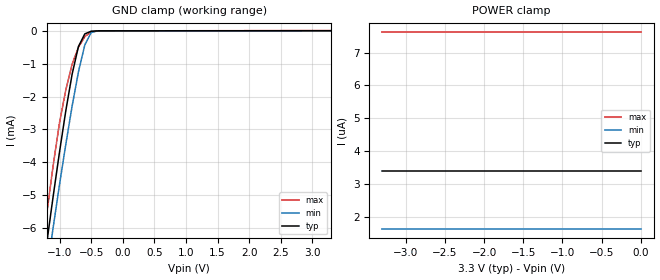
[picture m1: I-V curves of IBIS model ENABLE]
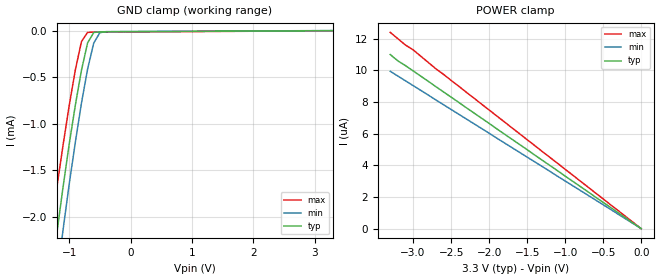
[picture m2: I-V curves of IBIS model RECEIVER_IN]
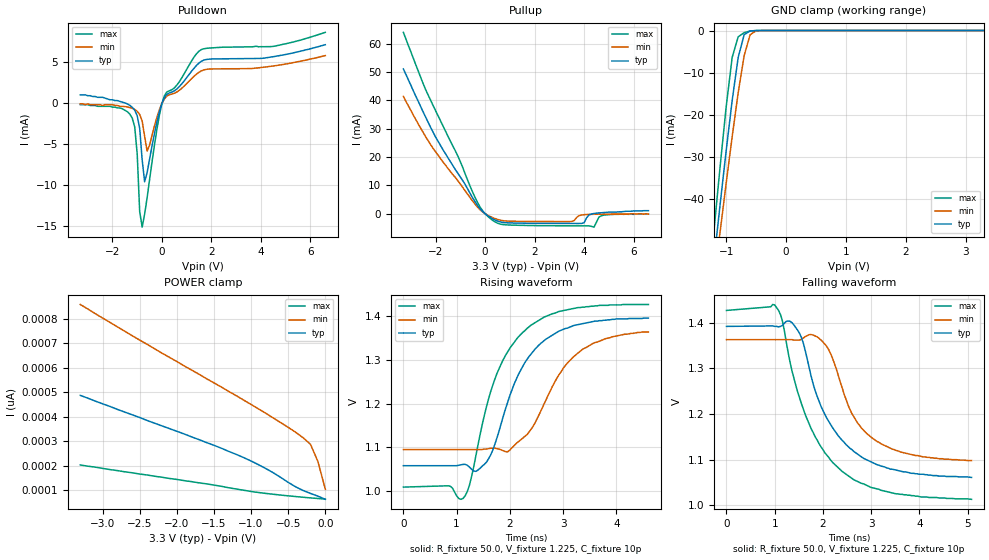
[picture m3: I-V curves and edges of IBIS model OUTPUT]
|   Texas Instruments Incorporated
|   Data Transmissions Products
|   IBIS Model for SN65LVDS108
|   38DBT TSSOP Package
[IBIS Ver]   3.2
[Comment char]   |_char
[File name]   lvds108a.ibs
[File Rev]   1.0
[Date]   14Apr00
[Source]   File originated at Texas Instruments Incorporated.
   Data Transmission Products Group
|   This model was updated to provide C_comp, mins and maxs 21Feb03
[Notes]
[Disclaimer]
(C) Copyright Texas Instruments Incorporated 2000
   All rights reserved
  Texas Instruments Incorporated hereby grants the user of this IBIS
model a non-exclusive, nontransferable license to use this IBIS model
under the following terms.  Before using this IBIS model, the user
should read this license.  If the user does not accept these terms,
the IBIS model should be returned to Texas Instruments within 30 days.
  The user is granted this license only to use the IBIS model and
is not granted rights to sell, load, rent, lease or license the IBIS
model in whole or in part, or in modified form to anyone other than
user.  User may modify the IBIS model to suit its specific applications
but rights to derivative works and such modifications shall belong to
Texas Instruments.
  This IBIS model is provided on an "AS IS" basis and Texas Instruments
makes absolutely no warranty with respect to the information contained
herein.  TEXAS INSTRUMENTS DISCLAIMS AND CUSTOMER WAIVES ALL WARRANTIES,
EXPRESS OR IMPLIED, INCLUDING WARRANTIES OF MERCHANTABILITY OR FITNESS
FOR A PARTICULAR PURPOSE. The entire risk as to quality and performance
is with the Customer. ACCORDINGLY, IN NO EVENT SHALL THE COMPANY BE LIABLE
FOR ANY DAMAGES, WHETHER IN CONTRACT OR TORT,INCLUDING ANY LOST PROFITS
OR OTHER INCIDENTAL, CONSEQUENTIAL, EXEMPLARY, OR PUNITIVE DAMAGES ARISING
OUT OF THE USE OR APPLICATION OF THE IBIS model provided in this package.
Further, Texas Instruments reserves the right to discontinue or make changes
without notice to any product herein to improve reliability, function, or
design. Texas Instruments does not convey any license under patent rights
or any other intellectual property rights, including those of third parties.
Contact Texas Instruments at ATTN:DATA TRANSMISSIONS
[Copyright]   Copyright 2000, Texas Instruments, All Rights Reserved
[Component]   LVDS108DBT
[Manufacturer]  Texas Instruments Incorporated
[Package]
|   typ   min   max
R_pkg   0.040   0.035   0.047
L_pkg   2.433nH   1.956nH   3.508nH
C_pkg   0.451pF   0.362pF   0.635pF
[Pin]   signal_name   model_name   R_pin   L_pin   C_pin
1   GND   GND   0.047   3.508n   0.598p
2   VCC   POWER   0.047   3.231n   0.634p
3   GND   GND   0.046   2.932n   0.570p
4   NC   NC
5   ENM   ENABLE   0.035   2.103n   0.387p
6   ENA   ENABLE   0.036   2.005n   0.369p
7   ENB   ENABLE   0.035   1.956n   0.365p
8   ENC   ENABLE   0.036   1.965n   0.364p
9   END   ENABLE   0.036   1.965n   0.363p
10   A   RECEIVER_IN   0.036   1.974n   0.362p
11   B   RECEIVER_IN   0.036   1.965n   0.362p
12   ENE   ENABLE   0.036   1.965n   0.364p
13   ENF   ENABLE   0.036   1.956n   0.365p
14   ENG   ENABLE   0.036   2.005n   0.369p
15   ENH   ENABLE   0.035   2.102n   0.387p
16   NC   NC
17   GND   GND   0.046   2.932n   0.570p
18   VCC   POWER   0.047   3.231n   0.634p
19   GND   GND   0.047   3.508n   0.598p
20   NC   NC
21   NC   NC
22   HZ   OUTPUT   0.046   2.932n   0.570p
23   HY   OUTPUT   0.043   2.459n   0.458p
24   GZ   OUTPUT   0.035   2.103n   0.387p
25   GY   OUTPUT   0.036   2.005n   0.369p
26   FZ   OUTPUT   0.035   1.956n   0.365p
27   FY   OUTPUT   0.036   1.965n   0.364p
28   EZ   OUTPUT   0.036   1.965n   0.363p
29   EY   OUTPUT   0.036   1.974n   0.363p
30   DZ   OUTPUT   0.036   1.965n   0.362p
31   DY   OUTPUT   0.036   1.965n   0.364p
32   CZ   OUTPUT   0.036   1.956n   0.365p
33   CY   OUTPUT   0.036   2.004n   0.369p
34   BZ   OUTPUT   0.035   2.102n   0.387p
35   BY   OUTPUT   0.043   2.459n   0.458p
36   AZ   OUTPUT   0.046   2.932n   0.570p
37   AY   OUTPUT   0.047   3.231n   0.635p
38   NC   NC
[Diff_pin]   inv_pin   vdiff   tdelay_typ   tdelay_min   tdelay_max
| The 'A' pin is Diff_pin and the 'B' pin is the inv_pin
10   11   0.100   0 0 0
23   22   0.000   0 0 0
25   24   0.000   0 0 0
27   26   0.000   0 0 0
29   28   0.000   0 0 0
31   30   0.000   0 0 0
33   32   0.000   0 0 0
35   34   0.000   0 0 0
37   36   0.000   0 0 0
| Models and submodels in the file (3): ENABLE (Input), RECEIVER_IN (Input), OUTPUT (3-state)
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|   Enable Model
[Model]   ENABLE
Model_type   Input
|Signals   ENM,ENA,ENB,ENC,END,ENE,ENF,ENG,ENH
Vinh = 2.0
Vinl = 0.8
|   typ   min   max
C_comp   1.10pF   1.02pF   1.21pF
|   typ   min   max
[Temperature Range]   25.0   -40   85
[Voltage range]   3.3V   3.0V   3.6V
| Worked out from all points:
|   GND clamp passes 1 mA (typ) near -0.76 V on its own axis
[GND_clamp]
|Voltage  I(typ)   I(min)   I(max)
-3.3V     -42.9mA    -42.4mA    -44.1mA
-1.3V     -7.87mA    -8.69mA    -7.06mA
-1.2V     -6.42mA    -7.31mA    -5.53mA
-1.1V     -5.02mA    -5.97mA    -4.08mA
-1V       -3.68mA    -4.67mA    -2.79mA
-900mV    -2.42mA    -3.44mA    -1.79mA
-800mV    -1.31mA    -2.28mA    -1.01mA
-700mV    -472uA     -1.24mA    -495uA
-600mV    -93.4uA    -429uA     -177uA
-500mV    -12.6uA    -53.4uA    -28.7uA
-400mV    -2.23uA    -3.52uA    -4.22uA
3.3V      3.38uA     1.63uA     7.62uA
[Power_clamp]
| Note that the[POWER_clamp]voltage table is referenced to Vcc
| and is calculated using Vtable=Vcc - Vmeasured.
|Voltage  I(typ)   I(min)   I(max)
-3.3V     3.38uA     1.63uA     7.62uA
-3.2V     3.38uA     1.63uA     7.62uA
-3.1V     3.38uA     1.63uA     7.62uA
0V        3.38uA     1.63uA     7.62uA
|   Receiver Input MODEL
[Model]   RECEIVER_IN
Model_type   Input
|Signals   A,B
Vinh = 2.0
Vinl = 0.8
|   typ   min   max
C_comp   1.18pF   1.14pF   1.21pF
|   typ   min   max
[Temperature Range]   25.0   -40   85
[Voltage range]   3.3V   3.0V   3.6V
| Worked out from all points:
|   GND clamp passes 1 mA (typ) near -0.95 V on its own axis
[GND_clamp]
|Voltage  I(typ)   I(min)   I(max)
-3.3V     -18.2mA    -19.6mA    -16.6mA
-1.3V     -2.68mA    -3.2mA     -2.16mA
-1.2V     -2.17mA    -2.66mA    -1.68mA
-1.1V     -1.68mA    -2.14mA    -1.23mA
-1V       -1.22mA    -1.65mA    -806uA
-900mV    -802uA     -1.2mA     -423uA
-800mV    -426uA     -779uA     -118uA
-700mV    -132uA     -413uA     -18.5uA
-600mV    -19.8uA    -134uA     -15.8uA
-500mV    -12.8uA    -21.9uA    -15.4uA
-400mV    -12.3uA    -10.7uA    -15uA
3.3V      7.23pA     904nA      -1.13uA
[Power_clamp]
| Note that the[POWER_clamp]voltage table is referenced to Vcc
| and is calculated using Vtable=Vcc - Vmeasured.
|Voltage  I(typ)   I(min)   I(max)
-3.3V     11uA       9.94uA     12.4uA
-3.2V     10.6uA     9.64uA     12uA
-3.1V     10.3uA     9.34uA     11.6uA
-3V       9.97uA     9.04uA     11.3uA
-2.7V     8.97uA     8.13uA     10.1uA
0V        7.23pA     7.89pA     8.43pA
|   Driver Output  MODEL
[Model]   OUTPUT
Model_type   3-state
| Signals   AY,AZ,BY,BZ,CY,CZ,DY,DZ,EY,EZ,FY,FZ,GY,GZ,HY,HZ
Vmeas = 1.2V   |Reference voltage for timing measurements
Cref = 10pF   |Timing specification test load capacitance value
Rref = 50   |Note: 50 Ohm load; single ended configuration
Vref = 1.20V   |Timing specification test load voltage
| variable   typ   min   max
C_comp   3.66pF   3.56pF   3.92pF
|   typ   min   max
[Temperature Range]   25.0   -40   85
[Voltage range]   3.3V   3.0V   3.6V
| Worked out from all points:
|   slope of the pulldown table from 0 to 0.495 V, typ, clamps not added: 326 ohm
|   slope of the pullup table from 0 to 0.495 V, typ, clamps not added: 192 ohm
|   GND clamp passes 1 mA (typ) near -0.70 V on its own axis
|   rising waveform, R_fixture 50.0, V_fixture 1.225, C_fixture 10p: 20-80 % time 733ps typ, 783ps min, 719ps max; typ from 1.06 V to 1.4 V
|   falling waveform, R_fixture 50.0, V_fixture 1.225, C_fixture 10p: 20-80 % time 875ps typ, 740ps min, 923ps max; typ from 1.39 V to 1.06 V
[Pulldown]
|Voltage  I(typ)   I(min)   I(max)
-3.3V     1mA        -100uA     -200uA
-1.7V     200uA      -400uA     -600uA
-1.2V     -520uA     -650uA     -1.85mA
-1.1V     -880uA     -790uA     -2.94mA
-1V       -1.55mA    -1.01mA    -6.24mA
-900mV    -3.1mA     -1.4mA     -13.3mA
-800mV    -6.95mA    -2.21mA    -15.2mA
-700mV    -9.64mA    -4.09mA    -13.6mA
-600mV    -8.52mA    -5.89mA    -11.6mA
0V        -34.7uA    -30.8uA    -40.1uA
1.4V      4.62mA     3.55mA     6.05mA
6.6V      7.14mA     5.81mA     8.66mA
[Pullup]
| Note that the[Pullup]voltage table is referenced to Vcc
| and is calculated using Vtable=Vcc - Vmeasured.
|Voltage  I(typ)   I(min)   I(max)
-3.3V     51.1mA     41.4mA     64mA
-2.4V     34.1mA     27.2mA     43.8mA
-1.7V     22.6mA     18.3mA     31mA
-1.1V     14.3mA     11.7mA     20.4mA
-300mV    2.89mA     2.33mA     3.94mA
300mV     -1.72mA    -1.33mA    -2.27mA
800mV     -3.13mA    -2.51mA    -3.87mA
3.5V      -3.4mA     -2.71mA    -4.24mA
3.9V      -3.4mA     -430uA     -4.25mA
4.4V      110uA      -160uA     -4.71mA
4.7V      370uA      -200uA     -670uA
6.6V      1.1mA      -100uA     -100uA
[GND_clamp]
| Outputs in High Impedance (off)
|Voltage  I(typ)   I(min)   I(max)
-3.3V     -347mA     -323mA     -383mA
-1.3V     -67.3mA    -71.1mA    -62mA
-1.2V     -54.1mA    -59.3mA    -46.9mA
-1.1V     -41.1mA    -47.6mA    -32.1mA
-1V       -28.5mA    -36.2mA    -18.1mA
-900mV    -16.6mA    -25.2mA    -6.38mA
-800mV    -6.42mA    -14.8mA    -1.5mA
-700mV    -997uA     -5.97mA    -506uA
-600mV    -101uA     -992uA     -108uA
-500mV    -8.6uA     -72.8uA    -9.14uA
3.3V      64pA       315pA      54.2pA
[POWER_clamp]
| Note that the [POWER_clamp] voltage table is referenced to Vcc
| and is calculated using Vtable = Vcc - Vmeasured.
| Outputs in Tri-state.
|Voltage  I(typ)   I(min)   I(max)
-3.3V     487pA      857pA      204pA
-2.5V     397pA      712pA      167pA
-1.5V     284pA      538pA      122pA
-1.2V     247pA      486pA      106pA
-800mV    189pA      414pA      88pA
-400mV    115pA      337pA      75.3pA
-300mV    100pA      315pA      72.5pA
-200mV    88pA       288pA      69.8pA
-100mV    77pA       218pA      67.4pA
0V        64pA       105pA      64.9pA
[Ramp]
|   Simulation with 100 ohm and 10pF loads.
|   typ   min   max
dV/dt_r   0.200/711ps   0.161/777ps   0.249/712ps
dV/dt_f   0.200/897ps   0.160/760ps   0.250/945ps
R_load = 50ohm
[Rising Waveform]
R_fixture = 50.0
V_fixture = 1.225
V_fixture_min = 1.229
V_fixture_max = 1.218
C_fixture = 10p
L_fixture = 0n
|   V(typ)  V(min)  V(max)
0s        1.058V     1.095V     1.009V
840ps     1.058V     1.095V     1.012V
1.16ns    1.061V     1.095V     989mV
1.44ns    1.052V     1.095V     1.129V
1.76ns    1.123V     1.097V     1.27V
2.08ns    1.245V     1.104V     1.34V
2.4ns     1.314V     1.142V     1.38V
3.2ns     1.379V     1.308V     1.418V
3.8ns     1.391V     1.349V     1.425V
4.6ns     1.396V     1.364V     1.427V
[Falling Waveform]
R_fixture = 50.0
V_fixture = 1.225
V_fixture_min = 1.229
V_fixture_max = 1.218
C_fixture = 10p
L_fixture = 0n
|   V(typ)  V(min)  V(max)
0s        1.392V     1.363V     1.427V
1ns       1.392V     1.363V     1.439V
1.16ns    1.394V     1.363V     1.404V
1.32ns    1.403V     1.363V     1.313V
1.52ns    1.376V     1.362V     1.234V
2ns       1.208V     1.358V     1.122V
2.4ns     1.142V     1.257V     1.074V
2.72ns    1.112V     1.18V      1.052V
3.2ns     1.086V     1.135V     1.033V
5.08ns    1.061V     1.098V     1.013V
